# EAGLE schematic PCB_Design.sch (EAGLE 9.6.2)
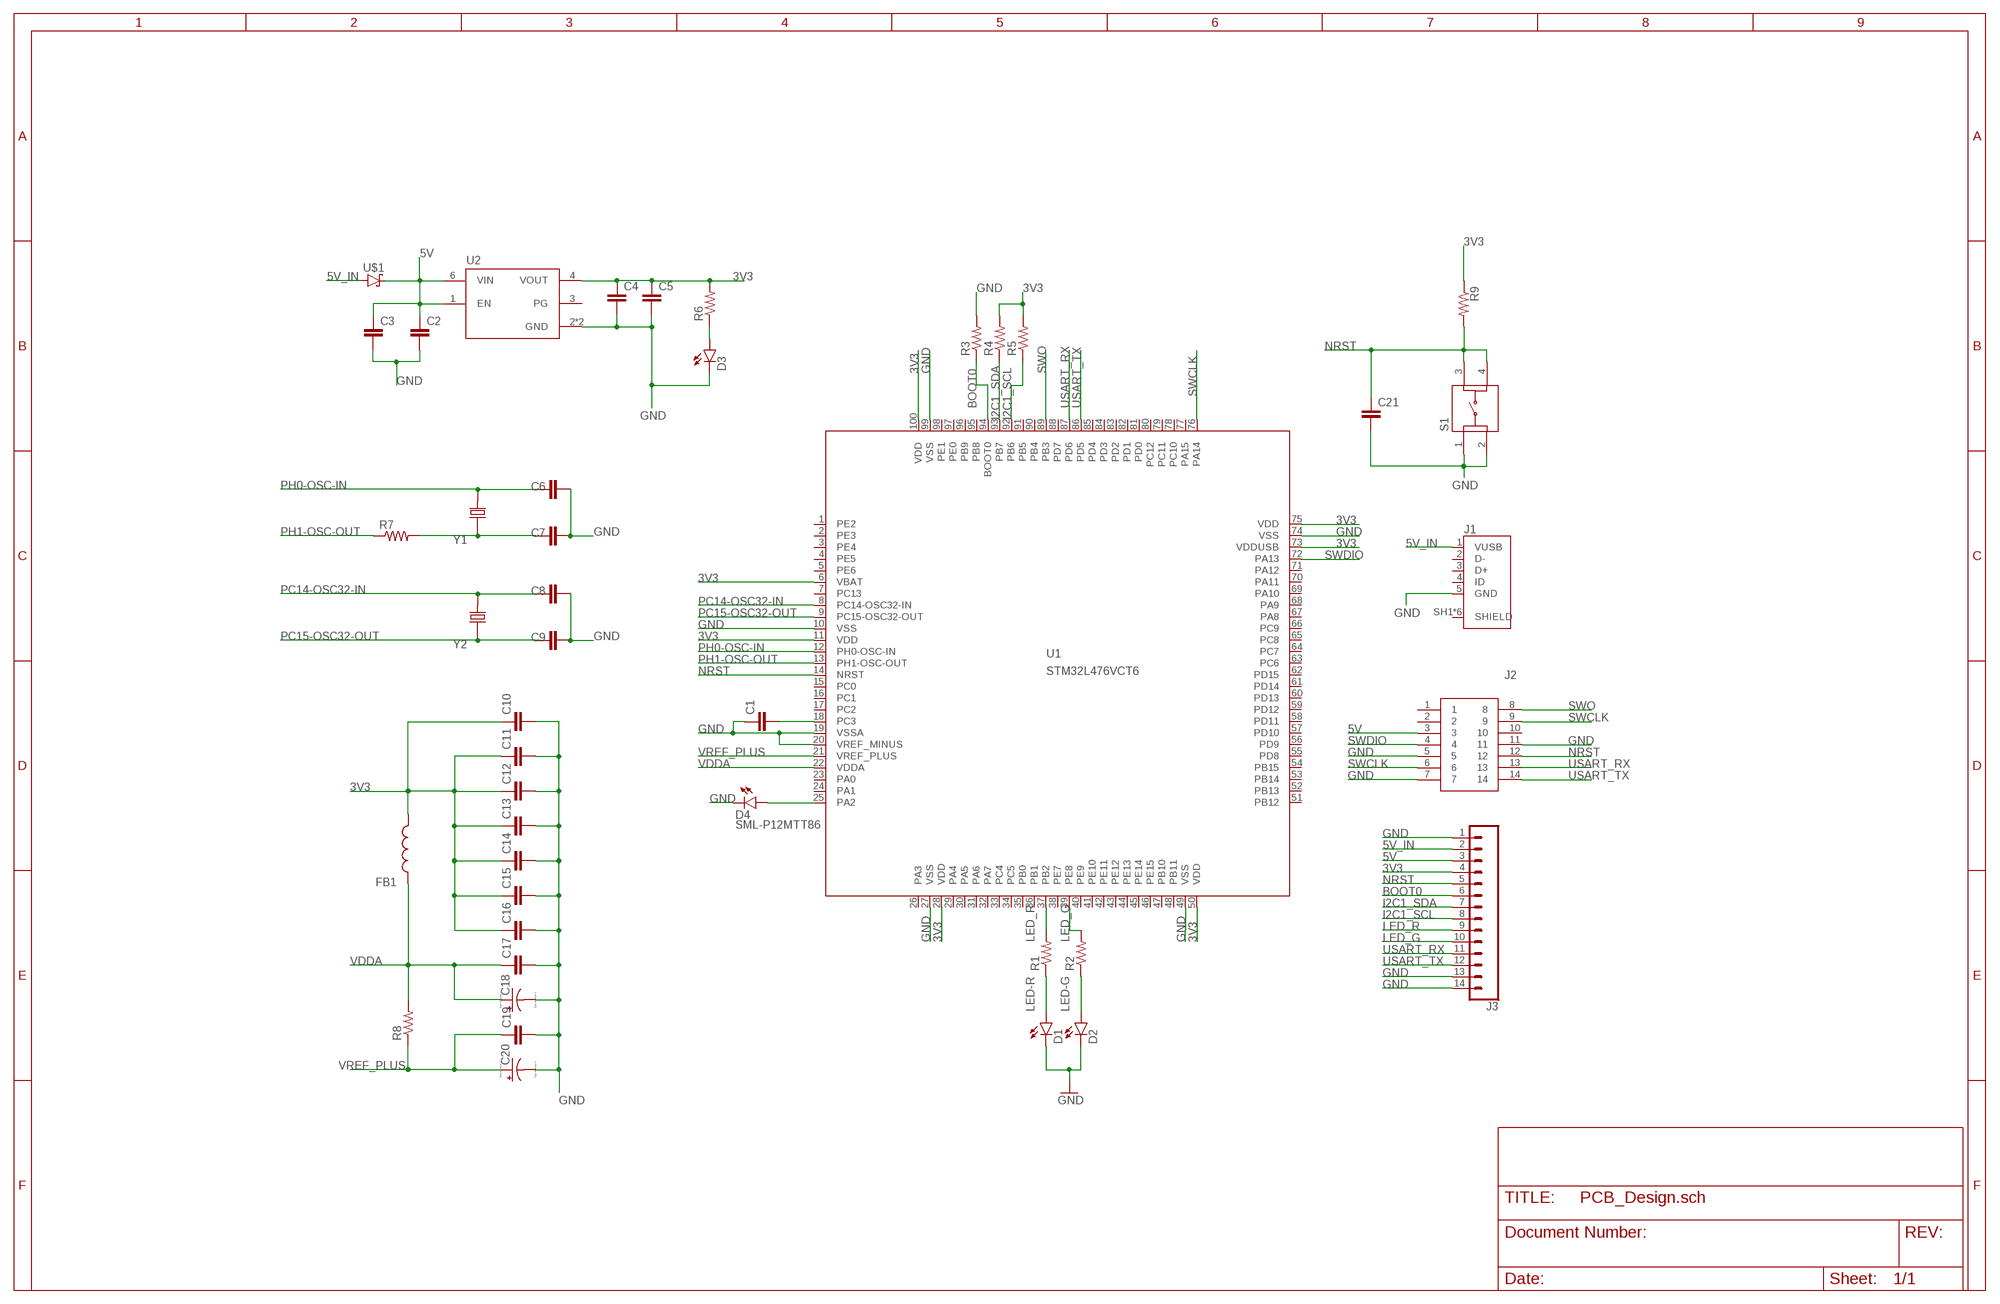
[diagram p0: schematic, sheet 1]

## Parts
C1  CC0603KRX5R7BB105  [CAPC1608X90]
C2  CC0603KRX5R7BB105  [CAPC1608X90]
C3  CC0603KRX5R7BB105  [CAPC1608X90]
C4  CC0603KRX5R7BB105  [CAPC1608X90]
C5  CC0603KRX5R7BB105  [CAPC1608X90]
C6  CC0402JRNPO9BN200  [CAPC1005X55N]
C7  CC0402JRNPO9BN200  [CAPC1005X55N]
C8  CC0402CRNPO9BN4R7  [CAPC1005X55N]
C9  CC0402CRNPO9BN4R7  [CAPC1005X55N]
C10  CC0603KRX5R7BB105  [CAPC1608X90]
C11  CC0402KRX7R7BB104  [CAPC1005X55N]
C12  CC0402KRX7R7BB104  [CAPC1005X55N]
C13  CC0402KRX7R7BB104  [CAPC1005X55N]
C14  CC0402KRX7R7BB104  [CAPC1005X55N]
C15  CC0402KRX7R7BB104  [CAPC1005X55N]
C16  CC0402KRX7R7BB104  [CAPC1005X55N]
C17  CC0402KRX7R7BB104  [CAPC1005X55N]
C18  TAJA105K016RNJ  [CAPPM3216X180N]
C19  CC0402KRX7R7BB104  [CAPC1005X55N]
C20  TAJA105K016RNJ  [CAPPM3216X180N]
C21  CC0402KRX7R7BB104  [CAPC1005X55N]
D1  SML-P12MTT86  [LED_SML-P11UTT86R]
D2  SML-P12MTT86  [LED_SML-P11UTT86R]
D3  SML-P12VTT86  [LED_SML-P11UTT86R]
D4  SML-P12MTT86  [LED_SML-P11UTT86R]
FB1  BK1608HS601-T  [BEADC1608X95N]
J1  10118192-0001LF  [AMPHENOL_10118192-0001LF]
J2  FTSH-107-01-L-DV-K-A  [FTSH10701LDVKA]
J3  CONN_14  [1X14]
R1  RC0402FR-071KL  [RESC1005X40N]
R2  RC0402FR-071KL  [RESC1005X40N]
R3  RC0402FR-071KL  [RESC1005X40N]
R4  RC0402FR-071KL  [RESC1005X40N]
R5  RC0402FR-071KL  [RESC1005X40N]
R6  RC0402FR-071KL  [RESC1005X40N]
R7  RC0402FR-071KL  [RESC1005X40N]
R8  RC0402FR-071KL  [RESC1005X40N]
R9  RC0402FR-071KL  [RESC1005X40N]
S1  LL3301FF065QJ  [LL3301FF065QJ]
U1  STM32L476VCT6  [LQFP100_14X14]
U2  LD39050PU33R  [SON95P300X300X100-7N]
U$1  STPS1L30A  [DIOM5226X223N]
Y1  ABLS-8.000MHZ-B2-T  [XTAL_ABLS-8.000MHZ-B2-T]
Y2  ECS-.327-12.5-12QS-TR  [XTAL_ECS-.327-12.5-12QS-TR]

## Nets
3V3: C4.1 C5.1 C10.1 C11.1 C12.1 C13.1 C14.1 C15.1 C16.1 FB1.2 J3.4 R4.2 R5.2 R6.2 R9.1 U1.6(VBAT) U1.11(VDD) U1.28(VDD) U1.50(VDD) U1.73(VDDUSB) U1.75(VDD) U1.100(VDD) U2.4(VOUT)
5V: C2.1 C3.1 J2.3 J3.3 U2.1(EN) U2.6(VIN) U$1.1(C)
5V_IN: J1.1(VUSB) J3.2 U$1.2(A)
BOOT0: J3.6 R3.1 U1.94(BOOT0)
GND: C1.1 C2.2 C3.2 C4.2 C5.2 C6.2 C7.2 C8.2 C9.2 C10.2 C11.2 C12.2 C13.2 C14.2 C15.2 C16.2 C17.2 C18.C(-) C19.2 C20.C(-) C21.2 D1.C D2.C D3.C D4.C J1.5(GND) J2.5 J2.7 J2.11 J3.1 J3.13 J3.14 R3.2 S1.1 S1.2 U1.10(VSS) U1.19(VSSA) U1.20(VREF_MINUS) U1.27(VSS) U1.49(VSS) U1.74(VSS) U1.99(VSS) U2.2(GND) U2.7(GND)
I2C1_SCL: J3.8 R5.1 U1.92(PB6)
I2C1_SDA: J3.7 R4.1 U1.93(PB7)
LED-G: D2.A R2.1
LED-R: D1.A R1.1
LED_G: J3.10 R2.2 U1.39(PE8)
LED_R: J3.9 R1.2 U1.37(PB2)
N$1: D4.A U1.25(PA2)
N$9: C7.1 R7.2 Y1.1
N$11: C1.2 U1.18(PC3)
N$14: D3.A R6.1
NRST: C21.1 J2.12 J3.5 R9.2 S1.3 S1.4 U1.14(NRST)
PC14-OSC32-IN: C8.1 U1.8(PC14-OSC32-IN) Y2.2
PC15-OSC32-OUT: C9.1 U1.9(PC15-OSC32-OUT) Y2.1
PH0-OSC-IN: C6.1 U1.12(PH0-OSC-IN) Y1.2
PH1-OSC-OUT: R7.1 U1.13(PH1-OSC-OUT)
SWCLK: J2.6 J2.9 U1.76(PA14)
SWDIO: J2.4 U1.72(PA13)
SWO: J2.8 U1.89(PB3)
USART_RX: J2.13 J3.11 U1.87(PD6)
USART_TX: J2.14 J3.12 U1.86(PD5)
VDDA: C17.1 C18.A(+) FB1.1 R8.2 U1.22(VDDA)
VREF_PLUS: C19.1 C20.A(+) R8.1 U1.21(VREF_PLUS)
Unconnected: J1.2(D-) J1.3(D+) J1.4(ID) J1.SH1(SHIELD) J1.SH2(SHIELD) J1.SH3(SHIELD) J1.SH4(SHIELD) J1.SH5(SHIELD) J1.SH6(SHIELD) J2.1 J2.2 J2.10 U1.1(PE2) U1.2(PE3) U1.3(PE4) U1.4(PE5) U1.5(PE6) U1.7(PC13) U1.15(PC0) U1.16(PC1) U1.17(PC2) U1.23(PA0) U1.24(PA1) U1.26(PA3) U1.29(PA4) U1.30(PA5) U1.31(PA6) U1.32(PA7) U1.33(PC4) U1.34(PC5) U1.35(PB0) U1.36(PB1) U1.38(PE7) U1.40(PE9) U1.41(PE10) U1.42(PE11) U1.43(PE12) U1.44(PE13) U1.45(PE14) U1.46(PE15) U1.47(PB10) U1.48(PB11) U1.51(PB12) U1.52(PB13) U1.53(PB14) U1.54(PB15) U1.55(PD8) U1.56(PD9) U1.57(PD10) U1.58(PD11) U1.59(PD12) U1.60(PD13) U1.61(PD14) U1.62(PD15) U1.63(PC6) U1.64(PC7) U1.65(PC8) U1.66(PC9) U1.67(PA8) U1.68(PA9) U1.69(PA10) U1.70(PA11) U1.71(PA12) U1.77(PA15) U1.78(PC10) U1.79(PC11) U1.80(PC12) U1.81(PD0) U1.82(PD1) U1.83(PD2) U1.84(PD3) U1.85(PD4) U1.88(PD7) U1.90(PB4) U1.91(PB5) U1.95(PB8) U1.96(PB9) U1.97(PE0) U1.98(PE1) U2.3(PG)

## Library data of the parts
C1-C5 C10 = ce-capstone:CC0603KRX5R7BB105: CAPACITOR CERAMIC, 1µF, 10V, X5R, 0603; Dielectric Characteristic:X5R; Capacitance:1µF; Capacitance Tolerance:± 10%; Voltage Rating:16V; Temperature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; DESCRIPTION: 1µF ±10% 16V Ceramic Capacitor X5R 0603 _1608 Metric_; DIGI-KEY_PART_NUMBER: 311-1444-1-ND; DIGI-KEY_PURCHASE_URL: https://www.digikey.com/product-detail/en/yageo/CC0603KRX5R7BB105/311-1444-1-ND/2833750?utm_source=snapeda&utm_medium=aggregator&utm_campaign=symbol; MF: Yageo; MP: CC0603KRX5R7BB105; PACKAGE: 0603 Yageo
C6 C7 = ce-capstone:CC0402JRNPO9BN200: CAPACITOR CERAMIC 20PF 50V, C0G, 0402; Dielectric Characteristic:C0G / NP0; Capacitance:20pF; Capacitance Tolerance:± 5%; Voltage Rating:50V; Capacitor Case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; DESCRIPTION: 20pF ±5% 50V Ceramic Capacitor C0G, NP0 0402 _1005 Metric_; DIGI-KEY_PART_NUMBER: 311-1417-1-ND; DIGI-KEY_PURCHASE_URL: https://www.digikey.com/product-detail/en/yageo/CC0402JRNPO9BN200/311-1417-1-ND/2833723?utm_source=snapeda&utm_medium=aggregator&utm_campaign=symbol; MF: Yageo; MP: CC0402JRNPO9BN200; PACKAGE: 0402 Yageo
C8 C9 = ce-capstone:CC0402CRNPO9BN4R7: 0402 4.7 pF 50 V ±0.25 pF Tolerance NP0 SMT Multilayer Ceramic Capacitor; DESCRIPTION: 4.7pF ±0.25pF 50V Ceramic Capacitor C0G, NP0 0402 _1005 Metric_; DIGI-KEY_PART_NUMBER: 311-1367-1-ND; DIGI-KEY_PURCHASE_URL: https://www.digikey.com/product-detail/en/yageo/CC0402CRNPO9BN4R7/311-1367-1-ND/2103151?utm_source=snapeda&utm_medium=aggregator&utm_campaign=symbol; MF: Yageo; MP: CC0402CRNPO9BN4R7; PACKAGE: 0402 Yageo
C11-C17 C19 C21 = ce-capstone:CC0402KRX7R7BB104: .1UF 16V 10% 0402; DESCRIPTION: 0.1µF ±10% 16V Ceramic Capacitor X7R 0402 _1005 Metric_; DIGI-KEY_PART_NUMBER: 311-1338-1-ND; DIGI-KEY_PURCHASE_URL: https://www.digikey.com/product-detail/en/yageo/CC0402KRX7R7BB104/311-1338-1-ND/2103122?utm_source=snapeda&utm_medium=aggregator&utm_campaign=symbol; MF: Yageo; MP: CC0402KRX7R7BB104; PACKAGE: 0402 Yageo
C18 C20 = ce-capstone:TAJA105K016RNJ: Capacitor tantalum TAJ 1206 1uF 16V AVX 1uF SMD Solid MnO2 Tantalum Electrolytic Capacitor, 16 V dc +/-10%, TAJ Series; ALLIED_NUMBER: 70474975; ALLIED_PRICE-STOCK: https://www.alliedelec.com/avx-taja105k016r/70474975/; DESCRIPTION: Capacitor tantalum TAJ 1206 1uF 16V AVX 1uF SMD Solid MnO2 Tantalum Electrolytic Capacitor, 16 V dc +/-10%, TAJ Series; HEIGHT: 1.8mm; MANUFACTURER_NAME: AVX; MANUFACTURER_PART_NUMBER: TAJA105K016RNJ; MOUSER_PART_NUMBER: 581-TAJA105K016RNJ; MOUSER_PRICE-STOCK: https://www.mouser.com/Search/Refine.aspx?Keyword=581-TAJA105K016R; RS_PART_NUMBER: 6992804P; RS_PRICE-STOCK: http://uk.rs-online.com/web/p/products/6992804P
D1 D2 D4 = ce-capstone:SML-P12MTT86: SML-P1 Series Red 0402 Clear 60 mcd 2 V Surface Mount PICOLED LED; AVAILABILITY: Unavailable; DESCRIPTION: Green 572nm LED Indication - Discrete 2V 0402 _1006 Metric_; MF: Rohm; MP: SML-P12MTT86; PACKAGE: 0402 Rohm; PRICE: None
D3 = ce-capstone:SML-P12VTT86: SML-P1 Series Red 0402 Clear 60 mcd 2 V Surface Mount PICOLED LED; AVAILABILITY: Unavailable; DESCRIPTION: Red 630nm LED Indication - Discrete 2V 0402 _1006 Metric_; MF: Rohm; MP: SML-P12VTT86; PACKAGE: 0402 Rohm; PRICE: None
FB1 = ce-capstone:BK1608HS601-T: Ferrite Chip Bead(Lead Free); DESCRIPTION: Ferrite Chip Bead(Lead Free); HEIGHT: 0.95mm; MANUFACTURER_NAME: Taiyo Yuden; MANUFACTURER_PART_NUMBER: BK1608HS601-T
J1 = ce-capstone:10118192-0001LF: Single Port 5 Contact Horizontal Right Angle Shielded Micro B USB 2.0 Connector; AVAILABILITY: Unavailable; DESCRIPTION: USB - micro B USB 2.0 Receptacle Connector 5 Position Surface Mount, Right Angle; MF: Amphenol ICC; MP: 10118192-0001LF; PACKAGE: None; PRICE: None
J2 = ce-capstone:FTSH-107-01-L-DV-K-A: Headers & Wire Housings .050" Micro Terminal Strip Source: Datasheet; DESCRIPTION: Headers & Wire Housings .050" Micro Terminal Strip; HEIGHT: 5.97mm; MANUFACTURER_NAME: SAMTEC; MANUFACTURER_PART_NUMBER: FTSH-107-01-L-DV-K-A; MOUSER_PART_NUMBER: 200-FTSH10701LDVKA; MOUSER_PRICE-STOCK: https://www.mouser.com/Search/Refine.aspx?Keyword=200-FTSH10701LDVKA
J3 = SparkFun-Connectors:CONN_14: Multi connection point. Often used as Generic Header-pin footprint for 0.1 inch spaced/style header connections On any of the 0.1 inch spaced packages, you can populate with these: Break Away Headers - Straight (PRT-00116) Break Away Male Headers - Right Angle (PRT-00553) Female Headers (PRT-00115)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
R1-R9 = ce-capstone:RC0402FR-071KL: RES SMD 510 OHM 1% 1/16W 0402; DESCRIPTION: 510 Ohms ±1% 0.063W, 1/16W Chip Resistor 0402 _1005 Metric_ Moisture Resistant Thick Film; DIGI-KEY_PART_NUMBER: 311-510LRCT-ND; DIGI-KEY_PURCHASE_URL: https://www.digikey.com/product-detail/en/yageo/RC0402FR-07510RL/311-510LRCT-ND/729579?utm_source=snapeda&utm_medium=aggregator&utm_campaign=symbol; MF: Yageo; MP: RC0402FR-07510RL; PACKAGE: 1005 Panasonic Electronic Components
S1 = ce-capstone:LL3301FF065QJ: Pushbutton Switches 50mA 12VDC F065 7.0mm J-Lead Source: Datasheet; DESCRIPTION: Pushbutton Switches 50mA 12VDC F065 7.0mm J-Lead; HEIGHT: 7.3mm; MANUFACTURER_NAME: E-Switch; MANUFACTURER_PART_NUMBER: LL3301FF065QJ; MOUSER_PART_NUMBER: 612-LL3301FF065QJ; MOUSER_PRICE-STOCK: https://www.mouser.com/Search/Refine.aspx?Keyword=612-LL3301FF065QJ
U1 = ce-capstone:STM32L476V*: STM32L476VX LQFP100 Datasheet STM32L476XX; FARNELL: 2518171; FLASH: 256kB; SRAM: 128kB
U2 = ce-capstone:LD39050PU33R: LD39050 Series 500 mA 3.3 V Fixed Low Noise LDO Voltage Regulator - DFN-6; AVAILABILITY: Unavailable; DESCRIPTION: Linear Voltage Regulator IC 1 Output 500mA 6-DFN _3x3_; MF: STMicroelectronics; MP: LD39050PU33R; PACKAGE: DFN-6 STMicroelectronics; PRICE: None
U$1 = ce-capstone:STPS1L30A
Y1 = ce-capstone:ABLS-8.000MHZ-B2-T: Crystal 8MHz Â±20ppm (Tol) Â±50ppm (Stability) 18pF FUND 80Ohm 2-Pin HC-49/US SMD T/R; AVAILABILITY: Unavailable; DESCRIPTION: 8MHz ±20ppm Crystal 18pF 80 Ohms HC-49/US; MF: Abracon LLC; MP: ABLS-8.000MHZ-B2; PACKAGE: HC-49/US Abracon LLC; PRICE: None
Y2 = ce-capstone:ECS-.327-12.5-12QS-TR: SMD CRYSTAL 32.768 KHz; AVAILABILITY: Unavailable; DESCRIPTION: 32.768kHz ±20ppm Crystal 12.5pF 90 kOhms 2-SMD, No Lead; MF: ECS Inc.; MP: ECS-.327-12.5-12QS-TR; PACKAGE: SMD-2 ECS International; PRICE: None

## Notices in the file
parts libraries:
SparkFun-Connectors: Licensing: Creative Commons ShareAlike 4.0 International - https://creativecommons.org/licenses/by-sa/4.0
